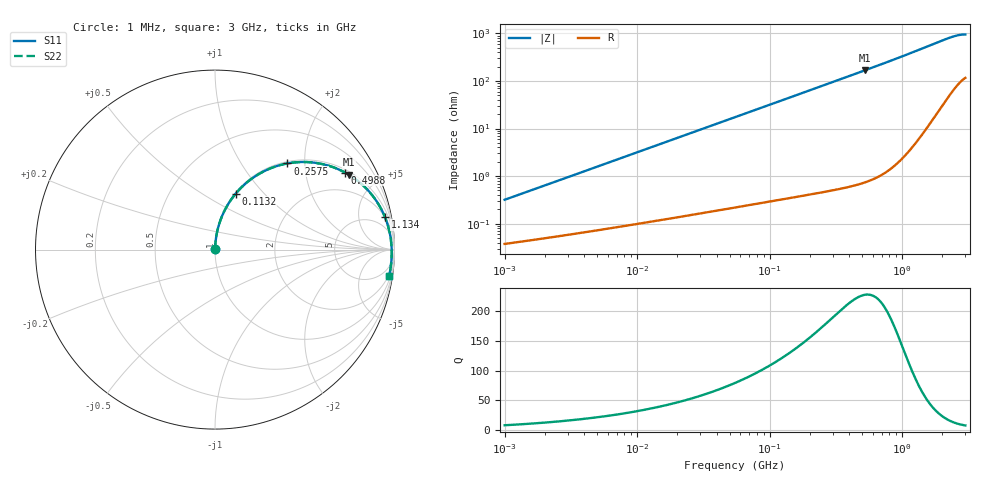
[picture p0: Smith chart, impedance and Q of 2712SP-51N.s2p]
# MHz  S  MA  R  50
!Freq  MagS11  AngS11  MagS21  AngS21  MagS12  AngS12  MagS22  AngS22
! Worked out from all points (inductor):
!   801 points, 1 MHz to 3 GHz, reference 50 ohm
!   read as one part in series: L = 50.3 nH near 1.041 MHz
!   highest Q = 227 at 524.4 MHz (marker M1), where L = 50.9 nH
!   S11 on the Smith chart (normalised r, x): 1 MHz: 1.00, +0.01; 113.2 MHz: 1.01, +0.71; 257.5 MHz: 1.03, +1.64; 498.8 MHz: 1.12, +3.31; 1.134 GHz: 2, +10; 3 GHz: 2, -13
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1  0.003152 83.0  0.9996 -0.2  0.9996 -0.2  0.003152 83.0
3.829105  0.012 86.2  0.9993 -0.7  0.9993 -0.7  0.012 86.2
14.51587  0.04537 85.9  0.9978 -2.6  0.9978 -2.6  0.04536 85.9
29.86408  0.09297 83.6  0.994 -5.4  0.994 -5.4  0.09296 83.6
55.02866  0.1695 79.3  0.9834 -9.9  0.9834 -9.9  0.1695 79.3
81.33854  0.2463 74.9  0.9667 -14.5  0.9667 -14.5  0.2462 74.9
113.2126  0.3334 69.6  0.9399 -19.9  0.9399 -19.9  0.3333 69.6
154.451  0.4345 63.3  0.8975 -26.3  0.8975 -26.3  0.4344 63.3
208.6098  0.546 55.8  0.8343 -33.8  0.8343 -33.8  0.5459 55.8
257.4635  0.6269 50.0  0.7755 -39.7  0.7755 -39.7  0.6268 50.0
302.2312  0.6869 45.3  0.7231 -44.4  0.7231 -44.4  0.6868 45.3
354.783  0.7432 40.5  0.6655 -49.2  0.6655 -49.2  0.743 40.5
416.4725  0.7939 35.8  0.6044 -54.0  0.6044 -54.0  0.7938 35.8
498.7844  0.843 30.6  0.5343 -59.2  0.5343 -59.2  0.8428 30.6
524.4091  0.8551 29.2  0.5149 -60.6  0.5149 -60.6  0.8549 29.2
640.7663  0.8964 23.9  0.4393 -65.9  0.4393 -65.9  0.8962 23.9
790.8254  0.9289 18.7  0.3658 -71.0  0.3658 -71.0  0.9287 18.7
1134.315  0.9638 10.9  0.2582 -78.5  0.2582 -78.5  0.9636 10.9
1610.776  0.9802 4.3  0.1776 -84.4  0.1776 -84.4  0.9799 4.3
2333.671  0.9848 -2.8  0.1191 -89.0  0.1191 -89.0  0.9847 -2.8
2685.098  0.9836 -5.8  0.1067 -90.2  0.1067 -90.2  0.9836 -5.8
3000  0.9813 -8.6  0.1033 -91.4  0.1033 -91.4  0.9815 -8.6
